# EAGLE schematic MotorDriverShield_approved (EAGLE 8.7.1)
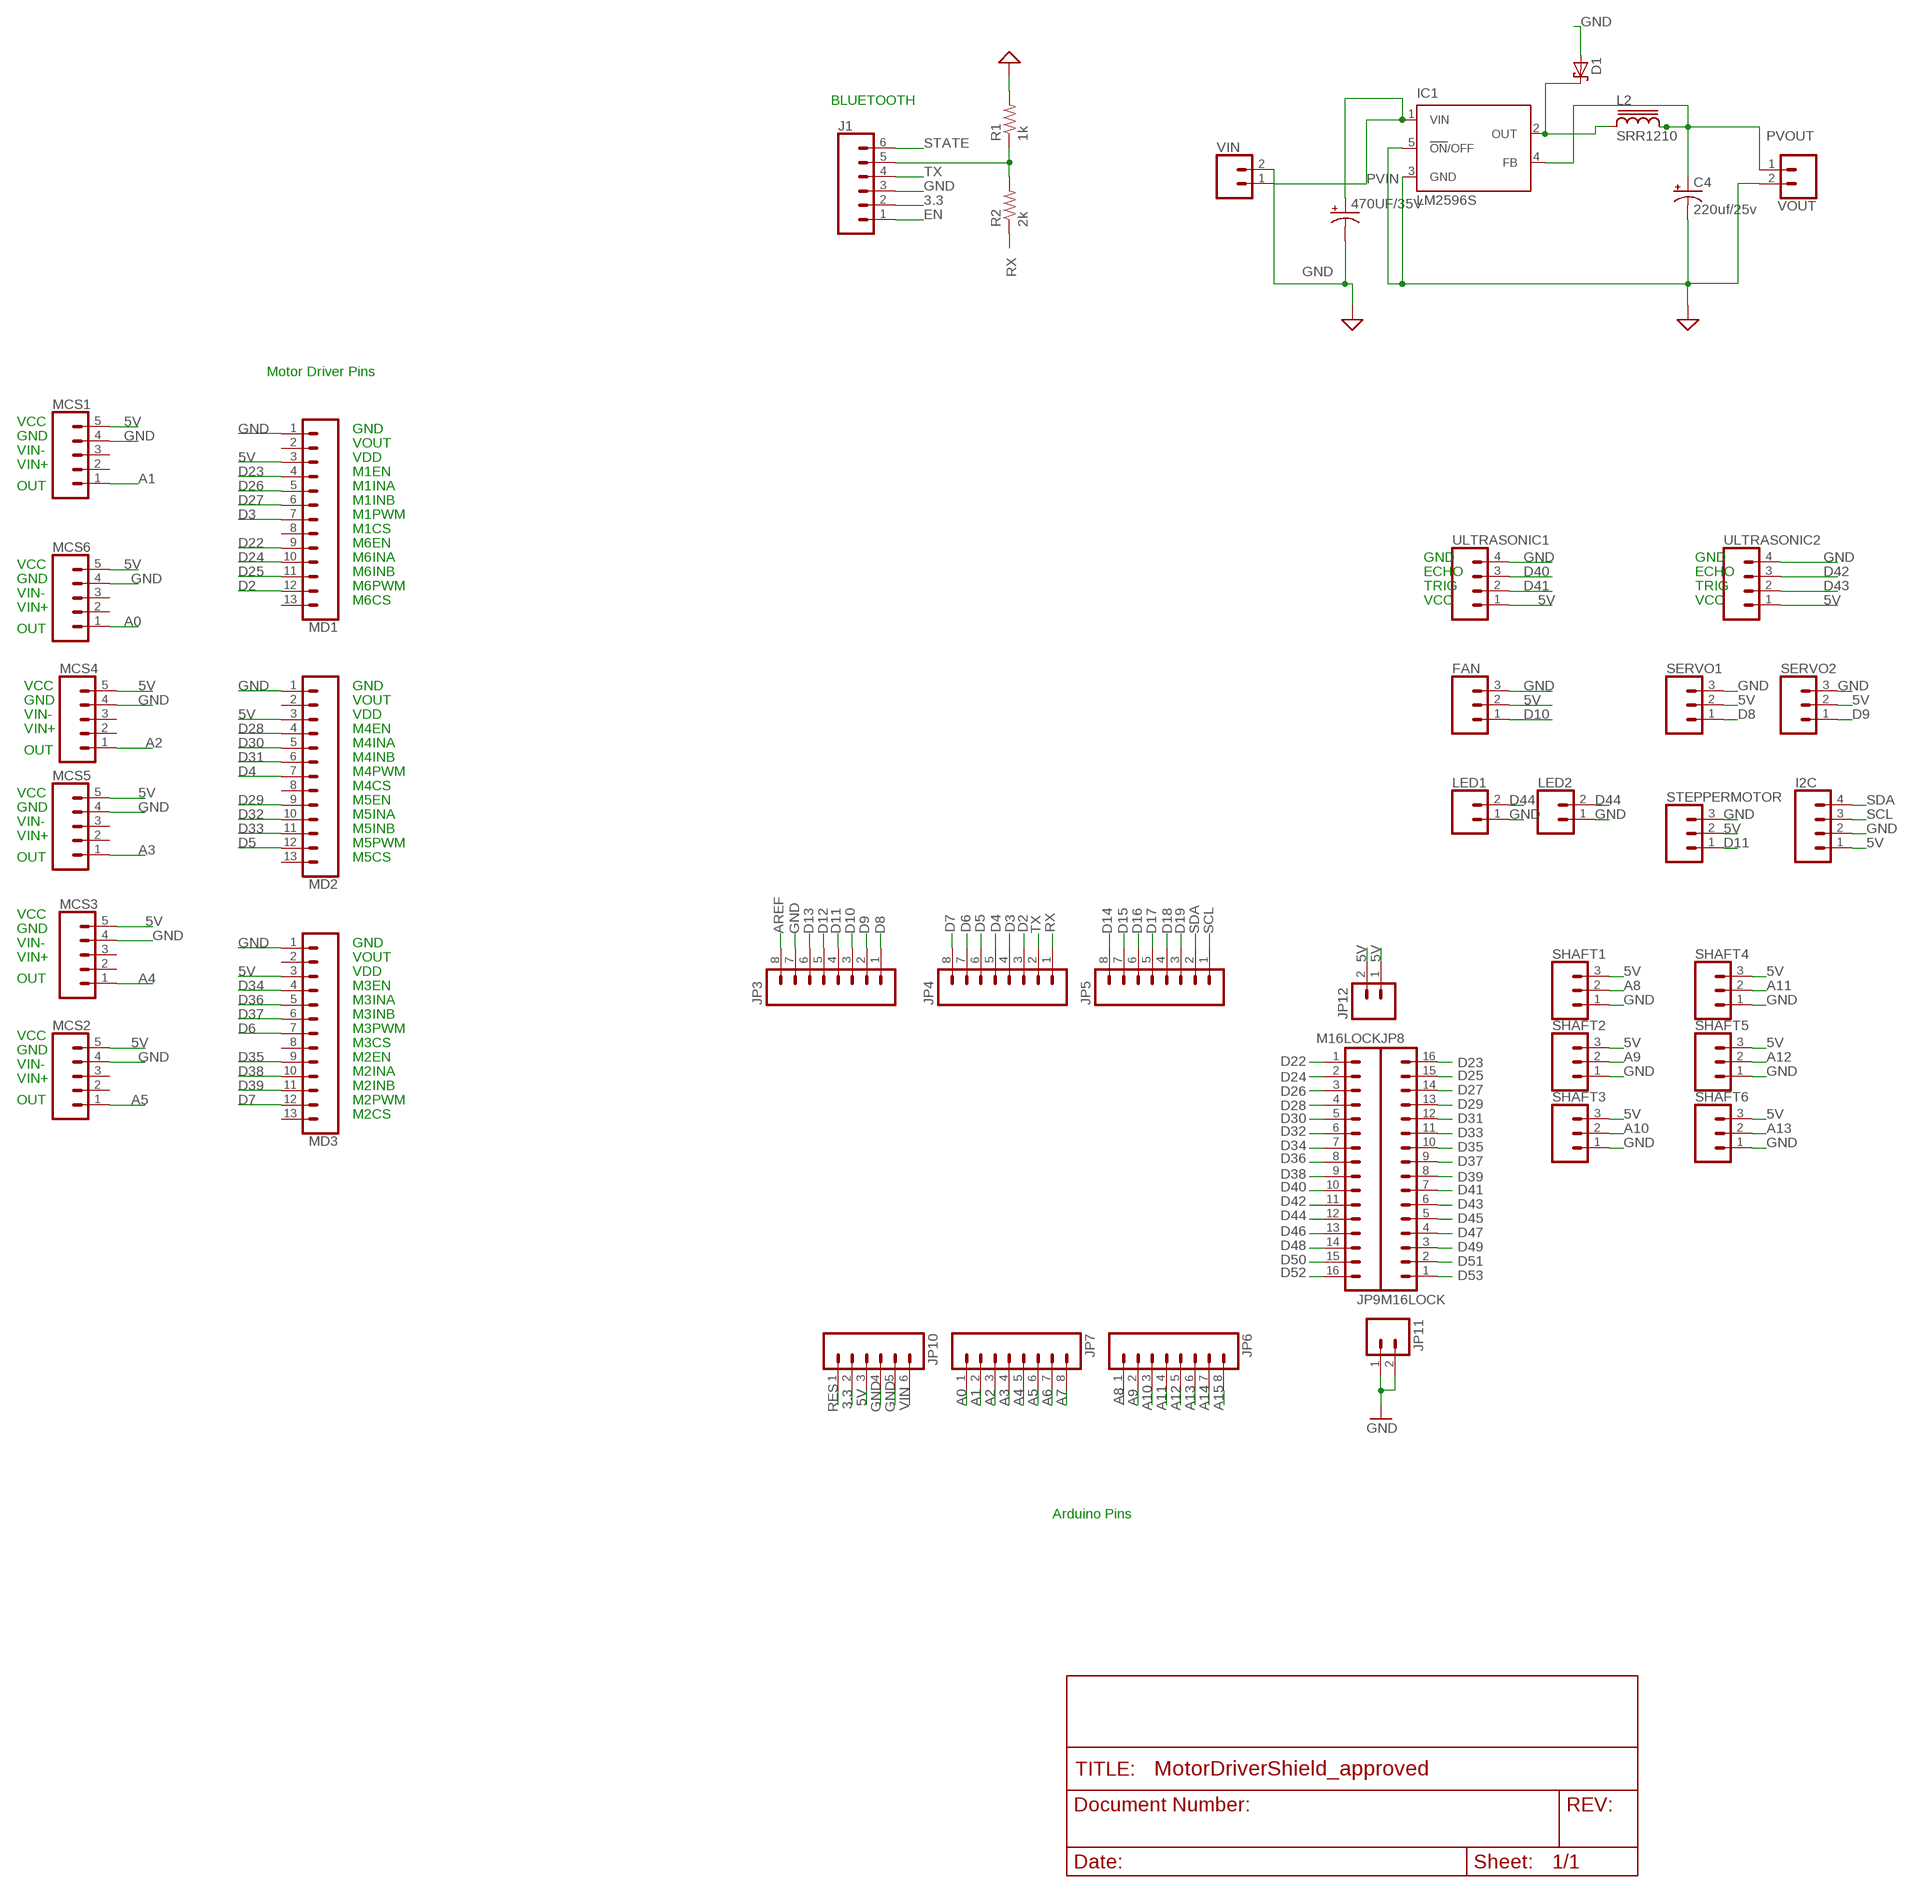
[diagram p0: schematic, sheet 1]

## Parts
470UF/35V  CPOLH13  [CPOL_PANASONIC_H13]
C4  220uf/25v  CPOLG  [CPOL_PANASONIC_G]
D1  SCHOTTKY-DIODESMC  [SMC]
FAN  CONN_03  [1X03]
I2C  CONN_04  [1X04]
IC1  LM2596S  [TO263-5]
J1  CONN_06LOCK  [1X06_LOCK]
JP3  M08LOCK  [1X08_LOCK]
JP4  M08LOCK  [1X08_LOCK]
JP5  M08LOCK  [1X08_LOCK]
JP6  M08LOCK  [1X08_LOCK]
JP7  M08LOCK  [1X08_LOCK]
JP8  M16LOCK  [1X16_LOCK]
JP9  M16LOCK  [1X16_LOCK]
JP10  M06LOCK  [1X06_LOCK]
JP11  M02LOCK  [1X02_LOCK]
JP12  M02LOCK  [1X02_LOCK]
L2  SRR1210  [SRR1210]
LED1  CONN_02LOCK  [1X02_LOCK]
LED2  CONN_02LOCK  [1X02_LOCK]
MCS1  CONN_05LOCK  [1X05_LOCK]
MCS2  CONN_05LOCK  [1X05_LOCK]
MCS3  CONN_05LOCK  [1X05_LOCK]
MCS4  CONN_05LOCK  [1X05_LOCK]
MCS5  CONN_05LOCK  [1X05_LOCK]
MCS6  CONN_05LOCK  [1X05_LOCK]
MD1  CONN_13  [1X13]
MD2  CONN_13  [1X13]
MD3  CONN_13  [1X13]
R1  1k  R-US_R0603  [R0603]
R2  2k  R-US_R0603  [R0603]
SERVO1  CONN_03LOCK  [1X03_LOCK]
SERVO2  CONN_03LOCK  [1X03_LOCK]
SHAFT1  CONN_03LOCK  [1X03_LOCK]
SHAFT2  CONN_03LOCK  [1X03_LOCK]
SHAFT3  CONN_03LOCK  [1X03_LOCK]
SHAFT4  CONN_03LOCK  [1X03_LOCK]
SHAFT5  CONN_03LOCK  [1X03_LOCK]
SHAFT6  CONN_03LOCK  [1X03_LOCK]
STEPPERMOTOR  CONN_03LOCK  [1X03_LOCK]
ULTRASONIC1  CONN_04  [1X04]
ULTRASONIC2  CONN_04  [1X04]
VIN  CONN_025MM  [SCREWTERMINAL-5MM-2]
VOUT  CONN_025MM  [SCREWTERMINAL-5MM-2]

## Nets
3.3: J1.2 JP10.2
5V: FAN.2 I2C.1 JP10.3 JP12.1 JP12.2 MCS1.5 MCS2.5 MCS3.5 MCS4.5 MCS5.5 MCS6.5 MD1.3 MD2.3 MD3.3 SERVO1.2 SERVO2.2 SHAFT1.3 SHAFT2.3 SHAFT3.3 SHAFT4.3 SHAFT5.3 SHAFT6.3 STEPPERMOTOR.2 ULTRASONIC1.1 ULTRASONIC2.1
A0: JP7.1 MCS6.1
A1: JP7.2 MCS1.1
A2: JP7.3 MCS4.1
A3: JP7.4 MCS5.1
A4: JP7.5 MCS3.1
A5: JP7.6 MCS2.1
A6: JP7.7
A7: JP7.8
A8: JP6.1 SHAFT1.2
A9: JP6.2 SHAFT2.2
A10: JP6.3 SHAFT3.2
A11: JP6.4 SHAFT4.2
A12: JP6.5 SHAFT5.2
A13: JP6.6 SHAFT6.2
A14: JP6.7
A15: JP6.8
AREF: JP3.8
D2: JP4.3 MD1.12
D3: JP4.4 MD1.7
D4: JP4.5 MD2.7
D5: JP4.6 MD2.12
D6: JP4.7 MD3.7
D7: JP4.8 MD3.12
D8: JP3.1 SERVO1.1
D9: JP3.2 SERVO2.1
D10: FAN.1 JP3.3
D11: JP3.4 STEPPERMOTOR.1
D12: JP3.5
D13: JP3.6
D14: JP5.8
D15: JP5.7
D16: JP5.6
D17: JP5.5
D18: JP5.4
D19: JP5.3
D22: JP9.1 MD1.9
D23: JP8.16 MD1.4
D24: JP9.2 MD1.10
D25: JP8.15 MD1.11
D26: JP9.3 MD1.5
D27: JP8.14 MD1.6
D28: JP9.4 MD2.4
D29: JP8.13 MD2.9
D30: JP9.5 MD2.5
D31: JP8.12 MD2.6
D32: JP9.6 MD2.10
D33: JP8.11 MD2.11
D34: JP9.7 MD3.4
D35: JP8.10 MD3.9
D36: JP9.8 MD3.5
D37: JP8.9 MD3.6
D38: JP9.9 MD3.10
D39: JP8.8 MD3.11
D40: JP9.10 ULTRASONIC1.3
D41: JP8.7 ULTRASONIC1.2
D42: JP9.11 ULTRASONIC2.3
D43: JP8.6 ULTRASONIC2.2
D44: JP9.12 LED1.2 LED2.2
D45: JP8.5
D46: JP9.13
D47: JP8.4
D48: JP9.14
D49: JP8.3
D50: JP9.15
D51: JP8.2
D52: JP9.16
D53: JP8.1
EN: J1.1
GND: 470UF/35V.- C4.- D1.A FAN.3 I2C.2 IC1.3(GND) IC1.5(!ON!/OFF) J1.3 JP3.7 JP10.4 JP10.5 JP11.1 JP11.2 LED1.1 LED2.1 MCS1.4 MCS2.4 MCS3.4 MCS4.4 MCS5.4 MCS6.4 MD1.1 MD2.1 MD3.1 R1.2 SERVO1.3 SERVO2.3 SHAFT1.1 SHAFT2.1 SHAFT3.1 SHAFT4.1 SHAFT5.1 SHAFT6.1 STEPPERMOTOR.3 ULTRASONIC1.4 ULTRASONIC2.4 VIN.2 VOUT.2 ; supply symbol labelled SUP
OUT: D1.C IC1.2(OUT) L2.1
PVIN: 470UF/35V.+ IC1.1(VIN) VIN.1
PVOUT: C4.+ IC1.4(FB) L2.2 VOUT.1
RES: JP10.1
RX: JP4.1 R2.1
RX0: J1.5 R1.1 R2.2
SCL: I2C.3 JP5.1
SDA: I2C.4 JP5.2
STATE: J1.6
TX: J1.4 JP4.2
VIN: JP10.6
Unconnected: MCS1.2 MCS1.3 MCS2.2 MCS2.3 MCS3.2 MCS3.3 MCS4.2 MCS4.3 MCS5.2 MCS5.3 MCS6.2 MCS6.3 MD1.2 MD1.8 MD1.13 MD2.2 MD2.8 MD2.13 MD3.2 MD3.8 MD3.13

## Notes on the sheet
- BLUETOOTH
- Motor Driver Pins
- VCC
- GND
- GND
- VOUT
- VIN-
- VDD
- VIN+
- M1EN
- OUT | M1INA
- M1INB
- M1PWM
- M1CS
- M6EN
- M6INA | GND | GND
- VCC
- M6INB | ECHO | ECHO
- GND
- M6PWM | TRIG | TRIG
- VIN-
- M6CS | VCC | VCC
- VIN+
- OUT
- VCC | GND
- GND | VOUT
- VIN- | VDD
- VIN+ | M4EN
- M4INA
- OUT
- M4INB
- M4PWM
- M4CS
- VCC
- M5EN
- GND
- M5INA
- VIN-
- M5INB
- VIN+
- M5PWM
- OUT | M5CS
- VCC
- GND
- VIN- | GND
- VIN+ | VOUT
- VDD
- OUT
- M3EN
- M3INA
- M3INB
- M3PWM
- VCC
- M3CS
- GND
- M2EN
- VIN-
- M2INA
- VIN+
- M2INB
- OUT | M2PWM
- M2CS
- Arduino Pins

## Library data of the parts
470UF/35V C4 = ELL-i-Passive:CPOL: Polarized Capacitor � common SMD and some through-hole ones
D1 = diode:SCHOTTKY-DIODE: Schottky Diode
FAN SERVO1 SERVO2 SHAFT1-SHAFT6 STEPPERMOTOR = SparkFun-Connectors:CONN_03: Multi connection point. Often used as Generic Header-pin footprint for 0.1 inch spaced/style header connections On any of the 0.1 inch spaced packages, you can populate with these: Break Away Headers - Straight (PRT-00116) Break Away Male Headers - Right Angle (PRT-00553) Female Headers (PRT-00115)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
I2C ULTRASONIC1 ULTRASONIC2 = SparkFun-Connectors:CONN_04: Multi connection point. Often used as Generic Header-pin footprint for 0.1 inch spaced/style header connections On any of the 0.1 inch spaced packages, you can populate with these: Break Away Headers - Straight (PRT-00116) Break Away Male Headers - Right Angle (PRT-00553) Female Headers (PRT-00115)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; PROD_ID: CONN-09696
IC1 = national-semiconductor:LM2596: SIMPLE SWITCHER® Power Converter 150 kHz 3A Step-Down Voltage Regulator Source: http://www.national.com/ds/LM/LM2596.pdf; MF: NATIONAL SEMICONDUCTOR; MPN: LM2596S-ADJ/NOPB; OC_FARNELL: 9494367; OC_NEWARK: 41K3842
J1 = SparkFun-Connectors:CONN_06: Multi connection point. Often used as Generic Header-pin footprint for 0.1 inch spaced/style header connections On any of the 0.1 inch spaced packages, you can populate with these: Break Away Headers - Straight (PRT-00116) Break Away Male Headers - Right Angle (PRT-00553) Female Headers (PRT-00115)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
JP3-JP7 = SparkFun:M08: Header 8 Standard 8-pin 0.1" header. Use with straight break away headers (SKU : PRT-00116), right angle break away headers (PRT-00553), swiss pins (PRT-00743), machine pins (PRT-00117), and female headers (PRT-00115).
JP8 JP9 = SparkFun:M16
JP10 = SparkFun:M06: Header 6 Standard 6-pin 0.1" header. Use with straight break away headers (SKU : PRT-00116), right angle break away headers (PRT-00553), swiss pins (PRT-00743), machine pins (PRT-00117), and female headers (PRT-00115). Molex polarized connector foot print use with SKU : PRT-08094 with associated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
JP11 JP12 = SparkFun:M02: Header 2
L2 = inductor-bourns:SRR1210: POWER INDUCTOR
LED1 LED2 = SparkFun-Connectors:CONN_02: Multi connection point. Often used as Generic Header-pin footprint for 0.1 inch spaced/style header connections
MCS1-MCS6 = SparkFun-Connectors:CONN_05: Multi connection point. Often used as Generic Header-pin footprint for 0.1 inch spaced/style header connections On any of the 0.1 inch spaced packages, you can populate with these: Break Away Headers - Straight (PRT-00116) Break Away Male Headers - Right Angle (PRT-00553) Female Headers (PRT-00115)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
MD1-MD3 = SparkFun-Connectors:CONN_13: Multi connection point. Often used as Generic Header-pin footprint for 0.1 inch spaced/style header connections On any of the 0.1 inch spaced packages, you can populate with these: Break Away Headers - Straight (PRT-00116) Break Away Male Headers - Right Angle (PRT-00553) Female Headers (PRT-00115)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
R1 R2 = audio amplifier example:R-US_: RESISTOR, American symbol
VIN VOUT = SparkFun-Connectors:CONN_02: Multi connection point. Often used as Generic Header-pin footprint for 0.1 inch spaced/style header connections; SF_SKU: PRT-08432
